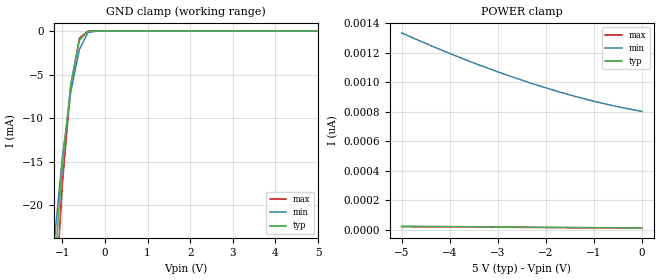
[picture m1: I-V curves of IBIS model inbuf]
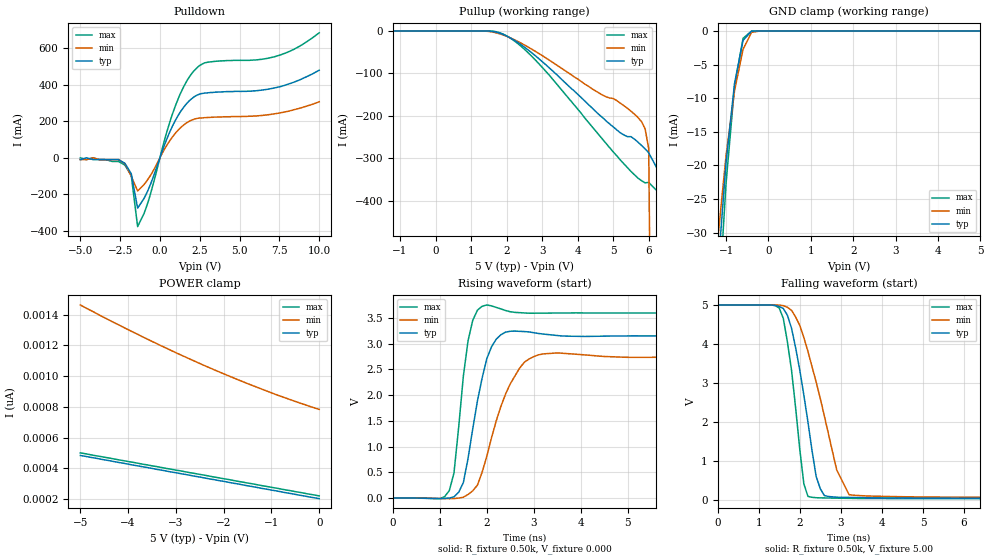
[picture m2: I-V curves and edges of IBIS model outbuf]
| IBIS file 41157p.ibs created by s2ibis2 version 1.0
| North Carolina State University Electronics Research Laboratory  1995
[IBIS ver]   2.1
[File name]   41157p.ibs
[File Rev]   0.1
[Date]   Friday, May 23, 1997
[Source]   IDT
[Notes]   1. Temp typ=25C, min=100C, max=0C 2. Ramp rates based on 500
   ohm load
[Copyright]   Copyright 1997, Integrated Device Technology, Inc.
[Disclaimer] Integrated Device Technology, Inc. ("IDT") hereby grants the
   user of this IBIS model a non-exclusive, nontransferable
   license to use this IBIS model under the following terms.
   The user is granted this license only to use the IBIS model
   and is not granted rights to sell, copy (except as needed to
   run the IBIS model), rent, lease or sub-license the IBIS model
   in whole or in part, or in modified form to anyone.
   The User may modify the IBIS model to suit its specific
   applications, but rights to derivative works and such
   modifications shall belong to IDT.
   This IBIS model is provided on an "AS IS" basis and IDT
   makes absolutely no warranty with respect to the information
   contained herein. IDT DISCLAIMS AND CUSTOMER WAIVES ALL
   WARRANTIES, EXPRESS AND IMPLIED, INCLUDING WARRANTIES OF
   MERCHANTABILITY AND FITNESS FOR A PARTICULAR PURPOSE. THE
   ENTIRE RISK AS TO QUALITY AND PERFORMANCE IS WITH THE
   USER ACCORDINGLY, IN NO EVENT SHALL IDT BE LIABLE
   FOR ANY DIRECT OR INDIRECT DAMAGES, WHETHER IN CONTRACT OR
   TORT, INCLUDING ANY LOST PROFITS OR OTHER INCIDENTAL,
   CONSEQUENTIAL, EXEMPLARY, OR PUNITIVE DAMAGES ARISING OUT OF
   THE USE OR APPLICATION OF THE IBIS model.  Further, IDT
   reserves the right to make changes without notice to any
   product herein to improve reliability, function, or design.
   IDT does not convey any license under patent rights or
   any other intellectual property rights, including those of
   third parties. IDT is not obligated to provide maintenance
   or support for the licensed IBIS model.
|   Component IDT54/74FCT157AT/CT/DT
[Component]   IDT54/74FCT157AT/CT/DT
[Manufacturer]   Integrated Device Technology Inc.
[Package]
| Following package parameters are for D20-1(CDIP), P20-1(DPIP) packages
|[Package]
|| variable   typ   min   max
|R_pkg   40.00m   30.00m   50.00m
|L_pkg   7.00nH   4.00nH   10.00nH
|C_pkg   0.60pF   0.50pF   0.70pF
| Following package parameters are for SO20-6(EIAJ), SO20-2(SOIC) packages
|[Package]
|| variable   typ   min   max
|R_pkg   25.00m   20.00m   30.00m
|L_pkg   3.50nH   2.10nH   6.50nH
|C_pkg   0.40pF   0.35pF   0.60pF
| Following package parameters are for SO20-8(QSOP), SO20-7(SSOP) packages
| variable   typ   min   max
R_pkg   20.00m   15.00m   25.00m
L_pkg   3.00nH   2.00nH   4.00nH
C_pkg   0.30pF   0.26pF   0.34pF
[Pin]  signal_name   model_name   R_pin   L_pin   C_pin
1   S   inbuf
2   I0A   inbuf
3   I1A   inbuf
4   ZA   outbuf
5   I0B   inbuf
6   I1B   inbuf
7   ZB   outbuf
8   GND   GND
9   ZD   outbuf
10   I1D   inbuf
11   I0D   inbuf
12   ZC   outbuf
13   I1C   inbuf
14   I0C   inbuf
15   EB   inbuf
16   VCC   POWER
| Models and submodels in the file (2): inbuf (Input), outbuf (3-state)
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| in   IN1   dummy_model
| oe   OE1   dummy_model
|   Model inbuf
[Model]   inbuf
Model_type   Input
Vinl =  0.800V
Vinh =  2.000V
C_comp   3.00pF   NA   NA
[Temperature Range]   25.00   100.00   0.000
[Voltage Range]   5.00V   4.50V   5.50V
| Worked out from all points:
|   GND clamp passes 1 mA (typ) near -0.59 V on its own axis
[GND_clamp]
| voltage   I(typ)   I(min)   I(max)
-5V       -67.15A    -63.94A    -68.24A
-1.2V     -28.45mA   -24.7mA    -34.05mA
-1V       -15.28mA   -14.53mA   -17.56mA
-800mV    -6.017mA   -6.948mA   -6.255mA
-600mV    -1.078mA   -2.117mA   -816uA
-400mV    -19.55uA   -178uA     -9.254uA
-200mV    -4.103nA   -287nA     -753pA
5V        12.62pA    835pA      10.26pA
[POWER_clamp]
| voltage   I(typ)   I(min)   I(max)
-5V       24.47pA    1.335nA    21.41pA
-4.3V     22.78pA    1.236nA    20pA
-3.6V     21.06pA    1.144nA    18.56pA
-3V       19.62pA    1.071nA    17.33pA
-2.3V     17.96pA    993pA      15.92pA
-1.7V     16.51pA    933pA      14.68pA
-1.1V     15.13pA    880pA      13.48pA
-600mV    13.99pA    842pA      12.44pA
0V        12.65pA    803pA      11.24pA
|   Model outbuf
[Model]   outbuf
Model_type   3-state
Polarity   Non-Inverting
Enable   Active-High
Vinl =  0.800V
Vinh =  2.000V
C_comp   3.00pF   NA   NA
[Temperature Range]   25.00   100.00   0.000
[Voltage Range]   5.00V   4.50V   5.50V
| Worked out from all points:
|   slope of the pulldown table from 0 to 0.75 V, typ, clamps not added: 4.5 ohm
|   GND clamp passes 1 mA (typ) near -0.54 V on its own axis
|   rising waveform, R_fixture 0.50k, V_fixture 0.000: 20-80 % time 380ps typ, 570ps min, 248ps max; typ from 0 V to 3.15 V
|   falling waveform, R_fixture 0.50k, V_fixture 5.00: 20-80 % time 455ps typ, 696ps min, 325ps max; typ from 5 V to 0.038 V
[Pulldown]
| voltage   I(typ)   I(min)   I(max)
-5V       -10mA      -10mA      0A
-2.2V     -30mA      -32mA      -40mA
-1.8V     -87mA      -101mA     -97mA
-1.4V     -276mA     -182mA     -377mA
-700mV    -168mA     -111mA     -230mA
300mV     73.42mA    49.04mA    101mA
900mV     193mA      127mA      268mA
1.5V      278mA      180mA      391mA
2.1V      331mA      210mA      473mA
3V        356mA      221mA      524mA
7.2V      383mA      241mA      554mA
10V       480mA      307mA      685mA
[Pullup]
| voltage   I(typ)   I(min)   I(max)
-5V       0A         0A         0A
1.8V      -4.879mA   -6.522mA   -3.82mA
2.8V      -57.68mA   -47.46mA   -67.5mA
4.8V      -212mA     -155mA     -265mA
5.1V      -233mA     -164mA     -294mA
5.7V      -262mA     -204mA     -347mA
5.9V      -278mA     -231mA     -358mA
6V        -287mA     -277mA     -357mA
6.4V      -350mA     -3.619A    -391mA
6.8V      -3.901A    -12.04A    -445mA
7.2V      -12.77A    -21.59A    -2.814A
10V       -84.2A     -93A       -72.68A
[GND_clamp]
| voltage   I(typ)   I(min)   I(max)
-5V       -84.19A    -80.05A    -85.71A
-1.2V     -36.11mA   -31.27mA   -43.35mA
-1V       -19.53mA   -18.47mA   -22.58mA
-800mV    -7.772mA   -8.883mA   -8.189mA
-600mV    -1.399mA   -2.708mA   -1.088mA
-400mV    -19.15uA   -190uA     -8.456uA
-200mV    -4.384nA   -314nA     -852pA
5V        202pA      835pA      192pA
[POWER_clamp]
| voltage   I(typ)   I(min)   I(max)
-5V       483pA      1.463nA    500pA
-4.3V     444pA      1.349nA    461pA
-3.7V     410pA      1.256nA    427pA
-3V       371pA      1.152nA    388pA
-2.4V     337pA      1.068nA    355pA
-1.7V     298pA      976pA      315pA
-900mV    253pA      879pA      271pA
0V        202pA      783pA      220pA
[Ramp]
| variable   typ   min   max
dV/dt_r   1.89/0.38n   1.64/0.57n   2.16/0.25n
dV/dt_f   2.98/0.46n   2.67/0.65n   3.28/0.35n
R_load = 0.50k
[Rising Waveform]
R_fixture = 0.50k
V_fixture = 0.000
| time   V(typ)   V(min)   V(max)
0s        0V         0V         0V
1.2ns     -572uV     -13.41mV   142mV
1.3ns     22.94mV    -10.15mV   487mV
1.5ns     301mV      15.44mV    2.373V
1.6ns     771mV      68.87mV    3.059V
1.9ns     2.334V     502mV      3.728V
2.1ns     2.941V     1.171V     3.736V
2.5ns     3.243V     2.222V     3.622V
3.1ns     3.2V       2.784V     3.595V
9.9ns     3.151V     2.741V     3.598V
[Falling Waveform]
R_fixture = 0.50k
V_fixture = 5.00
| time   V(typ)   V(min)   V(max)
0s        5V         5V         5V
1.5ns     4.963V     4.997V     4.924V
1.6ns     4.911V     4.984V     4.658V
1.8ns     4.404V     4.863V     3.328V
2.1ns     2.688V     4.167V     407mV
2.2ns     1.995V     3.806V     86.03mV
2.5ns     284mV      2.601V     48.72mV
2.9ns     65.32mV    766mV      40.84mV
3.2ns     59.64mV    130mV      36.49mV
9.9ns     37.52mV    56.99mV    27.47mV
